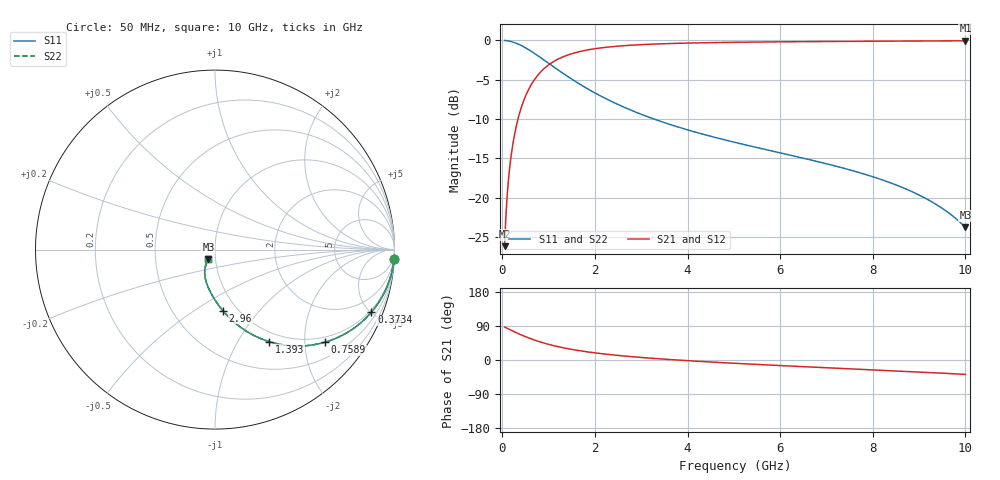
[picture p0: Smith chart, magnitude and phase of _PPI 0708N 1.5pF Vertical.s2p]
! S-Parameter data specifications (vertical orientation):
! Substrate: 40-mil Rogers 3003C, Substrate thickness, H=1.016mm, Dielectric constant, Er=3, Conductor thickness, T_mtl=0.043mm, Loss Tangent, Tand=0.003
! PCB Mounting Pad Footprint: Pad width, PadW=2.54mm , Pad length, PadL=0.51mm , Pad gap, PadG (edge-to-edge)=0.71mm , Reference planes=1.73mm apart
! Created Tue Jan 16 08:43:16 2018
# GHz S MA R 50
! 2 Port Network Data from SP1.SP block
! freq  magS11  angS11  magS21  angS21  magS12  angS12  magS22  angS22
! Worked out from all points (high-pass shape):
!   801 points, 50 MHz to 10 GHz, reference 50 ohm
!   highest |S21| = -0.06 dB at 10 GHz (marker M1); lowest = -26.2 dB at 50 MHz (marker M2)
!   |S21| within 3 dB of the highest: 1.014 GHz to end of sweep
!   lowest |S11| = -23.8 dB at 10 GHz (marker M3), VSWR 1.14, Z = 46.2 - j4.96 ohm
!   |S11| at or under -10 dB: 3.275 GHz to end of sweep
!   |S22| runs from -23.8 to 0.0 dB; largest |S21 - S12| = 0
!   S11 on the Smith chart (normalised r, x): 50 MHz: 1, -38; 373.4 MHz: 0.86, -5.05; 758.9 MHz: 0.86, -2.49; 1.393 GHz: 0.86, -1.36; 2.96 GHz: 0.86, -0.66; 10 GHz: 0.92, -0.10
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0.05  0.9988 -3.0  0.04919 87.0  0.04919 87.0  0.9988 -3.0
0.074875  0.9973 -4.5  0.07355 85.4  0.07355 85.4  0.9973 -4.5
0.1370625  0.991 -8.3  0.1338 81.7  0.1338 81.7  0.991 -8.3
0.1868125  0.9835 -11.2  0.1809 78.7  0.1809 78.7  0.9835 -11.2
0.224125  0.9765 -13.4  0.2155 76.6  0.2155 76.6  0.9765 -13.4
0.273875  0.9655 -16.3  0.2603 73.7  0.2603 73.7  0.9655 -16.3
0.373375  0.9386 -21.8  0.3448 68.2  0.3448 68.2  0.9386 -21.8
0.4604375  0.9109 -26.4  0.4124 63.6  0.4124 63.6  0.9109 -26.4
0.5475  0.8805 -30.7  0.4737 59.3  0.4737 59.3  0.8805 -30.7
0.7589375  0.802 -40.0  0.5968 50.0  0.5968 50.0  0.802 -40.0
1.069875  0.6913 -50.9  0.7219 39.0  0.7219 39.0  0.6913 -50.9
1.39325  0.5945 -59.6  0.8033 30.4  0.8033 30.4  0.5945 -59.6
1.716625  0.5174 -66.3  0.8548 23.6  0.8548 23.6  0.5174 -66.3
2.263875  0.4221 -74.8  0.9054 15.0  0.9054 15.0  0.4221 -74.8
2.960375  0.3425 -82.7  0.9382 7.1  0.9382 7.1  0.3425 -82.7
3.370812  0.3091 -86.5  0.9496 3.3  0.9496 3.3  0.3091 -86.5
5.025  0.2247 -98.3  0.9725 -8.8  0.9725 -8.8  0.2247 -98.3
6.691625  0.1729 -108.0  0.9825 -18.7  0.9825 -18.7  0.1729 -108.0
8.345812  0.1254 -116.8  0.989 -28.1  0.989 -28.1  0.1254 -116.8
9.278625  0.09397 -121.5  0.9919 -33.5  0.9919 -33.5  0.09397 -121.5
9.639313  0.08005 -123.1  0.9928 -35.7  0.9928 -35.7  0.08005 -123.1
10  0.06486 -124.5  0.9936 -37.9  0.9936 -37.9  0.06486 -124.5
